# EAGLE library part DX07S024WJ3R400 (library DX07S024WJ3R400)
Input/Output Connector, USB Type-C connector, 24 pos., Height: 10 mm, 2-row , Vertical-Receptacle Source: Datasheet
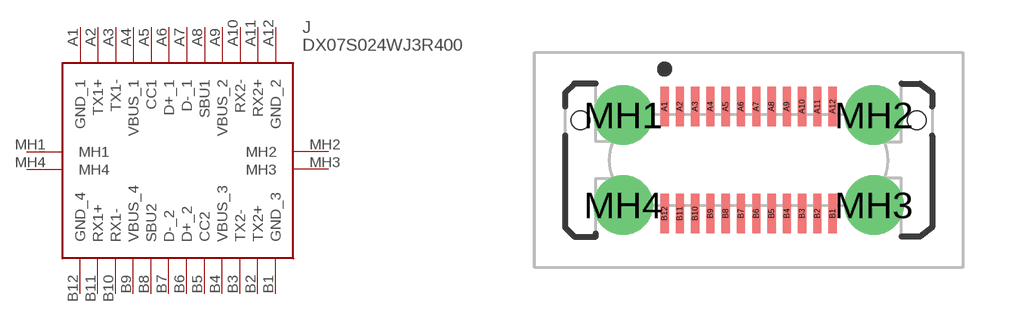
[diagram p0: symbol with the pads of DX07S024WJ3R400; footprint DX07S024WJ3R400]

Designator prefix J

## DX07S024WJ3R400 (Description: Input/Output Connector, USB Type-C connector, 24 pos., Height: 10 mm, 2-row , Vertical-Receptacle; Height: 10.2mm; Manufacturer_Name: JAE; Manufacturer_Part_Number: DX07S024WJ3R400; Mouser_Part_Number: 656-DX07S0024WJ3R400; Mouser_Price-Stock: https://www.mouser.co.uk/ProductDetail/JAE-Electronics/DX07S024WJ3R400?qs=Ps1sUSMe7kmTGGC30IqfqQ%3D%3D)  [DX07S024WJ3R400]
A1  GND_1
A2  TX1+
A3  TX1-
A4  VBUS_1
A5  CC1
A6  D+_1
A7  D-_1
A8  SBU1
A9  VBUS_2
A10  RX2-
A11  RX2+
A12  GND_2
B1  GND_3
B2  TX2+
B3  TX2-
B4  VBUS_3
B5  CC2
B6  D+_2
B7  D-_2
B8  SBU2
B9  VBUS_4
B10  RX1-
B11  RX1+
B12  GND_4
MH1  MH1
MH2  MH2
MH3  MH3
MH4  MH4

## Footprint DX07S024WJ3R400 (pad centres in mm)
DX07S024WJ3R400-1
smd 0.27 x 1.3: A1 -2.75,1.75; A2 -2.25,1.75; A3 -1.75,1.75; A4 -1.25,1.75; A5 -0.75,1.75; A6 -0.25,1.75; A7 0.25,1.75; A8 0.75,1.75; A9 1.25,1.75; A10 1.75,1.75; A11 2.25,1.75; A12 2.75,1.75; B1 2.75,-1.75; B2 2.25,-1.75; B3 1.75,-1.75; B4 1.25,-1.75; B5 0.75,-1.75; B6 0.25,-1.75; B7 -0.25,-1.75; B8 -0.75,-1.75; B9 -1.25,-1.75; B10 -1.75,-1.75; B11 -2.25,-1.75; B12 -2.75,-1.75
drill 1.3 pad 1.95: MH1 -4.1,1.47; MH2 4.1,1.47; MH3 4.1,-1.47; MH4 -4.1,-1.47
hole 0.6 at -5.5,1.3
hole 0.6 at 5.5,1.3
